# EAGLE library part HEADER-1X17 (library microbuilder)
Header 1x17
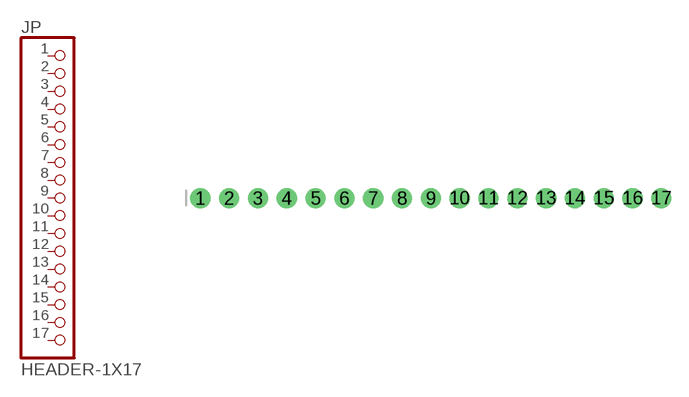
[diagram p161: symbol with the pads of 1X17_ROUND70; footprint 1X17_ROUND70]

Designator prefix JP

## HEADER-1X17  [1X17_ROUND70]
1  1  pas
2  2  pas
3  3  pas
4  4  pas
5  5  pas
6  6  pas
7  7  pas
8  8  pas
9  9  pas
10  10  pas
11  11  pas
12  12  pas
13  13  pas
14  14  pas
15  15  pas
16  16  pas
17  17  pas

## Footprint 1X17_ROUND70 (pad centres in mm)
drill 1 pad 1.778: 1 -20.32,0; 2 -17.78,0; 3 -15.24,0; 4 -12.7,0; 5 -10.16,0; 6 -7.62,0; 7 -5.08,0; 8 -2.54,0; 9 0,0; 10 2.54,0; 11 5.08,0; 12 7.62,0; 13 10.16,0; 14 12.7,0; 15 15.24,0; 16 17.78,0; 17 20.32,0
